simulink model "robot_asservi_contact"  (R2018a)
settings: Solver=VariableStepAuto  StartTime=0.0  StopTime=t(numel(t))  FixedStep=0.0001  RelTol=1e-3
model workspace: external: MATLAB File (data not in the file)
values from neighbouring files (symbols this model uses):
  D = [1500 1500 1000 0 0 0]    [TP_6Axes_main.m]
  dt = 0.01    [TP_6axes_trajectoire_polynomiale.m]    (also in TP_6axes_trajectoire_rectangulaire.m = 0.005)
  I = [0 0 0 0 0 0]    [TP_6Axes_main.m]
  mu = mu/3    [TP_6Axes_main.m]
  nx = length(ref)    [Jnum.m]    (also in TP_6axes_trajectoire_rectangulaire.m = 0.6)
  P = [16000 15000 14000 3000 3000 3000]    [TP_6Axes_main.m]
  q_targ = zeros(6,numel(p_targ(1,:)))    [TP_6axes_trajectoire_polynomiale.m]    (also in TP_6axes_trajectoire_rectangulaire.m)
  X = [T(1:3,4);Euler]    [MGD_6axes.m]    (also in TP_6axes_trajectoire_polynomiale.m = Trace_6axes_trajectoire(q_targ,p_targ,rob); TP_6axes_trajectoire_rectangulaire.m = Trace_6axes_trajectoire(q_targ,p_targ,rob); Trace_6axes.m = [0 0 0; Trace_6axes_trajectoire.m = [0 0 0)
undefined symbols (not defined in the file or in its folder): deg, kg, m, mm, N, rad, s, smiData, Y, Z
libraries: sm_lib x42, nesl_utility x23, Contact_Forces_Lib x1
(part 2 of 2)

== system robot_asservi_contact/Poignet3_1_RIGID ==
  ReferenceFrame : sm_lib/Frames and Transforms/Reference Frame
  Solid : sm_lib/Body Elements/Solid  InertiaType=Custom  Mass=smiData.Solid(2).mass  MassUnits=kg  CenterOfMass=smiData.Solid(2).CoM  CenterOfMassUnits=mm  MomentsOfInertia=smiData.Solid(2).MoI  MomentsOfInertiaUnits=kg*mm^2  ProductsOfInertia=smiData.Solid(2).PoI  ProductsOfInertiaUnits=kg*mm^2  DensityBased=on  Density=1000  DensityUnits=kg/m^3  DoExposeReferenceFrame=on  SerializedFrames=<Frames/>  GraphicType=FromGeometry  MarkerShape=Sphere  MarkerSize=10  GraphicVisPropType=SimpleVisualProperties  GraphicDiffuseColor=[0.4 1.0 1.0]  GraphicSpecularColor=[0.5 0.5 0.5 1.0]  GraphicAmbientColor=[0.15 0.15 0.15 1.0]  GraphicEmissiveColor=[0.0 0.0 0.0 1.0]  GraphicShininess=75  GraphicOpacity=smiData.Solid(2).opacity  GeometryShape=FromFile  RectangleSize=[1 1]  RectangleSizeUnits=m  BrickDimensions=[1 1 1]  BrickDimensionUnits=m  CylinderRadius=1  CylinderRadiusUnits=m  CylinderLength=1  CylinderLengthUnits=m  SphereRadius=1  SphereRadiusUnits=m  EllipsoidRadii=[1 1 1]  EllipsoidRadiiUnits=m  ExtrusionCrossSection=[1 1; -1 1; -1 -1; 1 -1]  ExtrusionCrossSectionUnits=m  ExtrusionLength=1  ExtrusionLengthUnits=m  PolygonNumSides=3  PolygonOuterRadius=1  PolygonOuterRadiusUnits=m  ExtGeomFileType=STL  ExtGeomFileName=Poignet3_Défaut_sldprt.STL  ExtGeomFileUnits=mm  RevolutionCrossSection=[1 1; 1 -1; 2 -1; 2 1]  RevolutionCrossSectionUnits=m  RevolutionExtent=Full  RevolutionAngle=180  RevolutionAngleUnits=deg
  Transform : sm_lib/Frames and Transforms/Rigid Transform  TranslationMethod=Cartesian  TranslationStandardOffset=0  TranslationLengthUnit=mm  TranslationStandardAxis=+Z  TranslationCartesianOffset=smiData.RigidTransform(6).translation  TranslationROffset=0  TranslationROffsetUnits=m  TranslationZOffset=0  TranslationZOffsetUnits=m  TranslationThetaOffset=0  TranslationThetaOffsetUnits=deg  RotationMethod=ArbitraryAxis  RotationAngleUnits=rad  RotationStandardAxis=+Z  RotationAngle=smiData.RigidTransform(6).angle  RotationArbitraryAxis=smiData.RigidTransform(6).axis  FollAlignAxisA=+X  BaseAlignAxisA=+Y  FollAlignAxisB=+Y  BaseAlignAxisB=+Z  RotationSequenceAxes=FollowerAxes  RotationSequence=XYX  RotationSequenceAngles=[0 0 0]  RotationSequenceAnglesUnits=deg  RotationMatrix=[1 0 0; 0 1 0; 0 0 1]
  F : PMIOPort  Side=Left
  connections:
  Solid/RConn1 -- ReferenceFrame/RConn1 -- Transform/LConn1
  Transform/RConn1 -- F/RConn1

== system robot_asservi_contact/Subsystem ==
  In1 : Inport
  Derivative : Derivative
  Derivative1 : Derivative
  Simulink-PS Converter6 : nesl_utility/Simulink-PS Converter  PhysicalDomain=network_engine_domain  SubClassName=ps_input  LeftPortType=input  RightPortType=output  PseudoPeriodic=off  Frequencies=[]  NoiseDistribution=none  NoiseParameters=[]  Unit=m  AffineConversion=off  FilteringAndDerivatives=provide  SimscapeFilterOrder=1  InputFilterTimeConstant=0.001  UdotUserProvided=2
  Conn1 : PMIOPort  Side=Right
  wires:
  In1/1 -> Derivative/1, Simulink-PS Converter6/1
  Derivative/1 -> Derivative1/1, Simulink-PS Converter6/2
  Derivative1/1 -> Simulink-PS Converter6/3
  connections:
  Simulink-PS Converter6/RConn1 -- Conn1/RConn1

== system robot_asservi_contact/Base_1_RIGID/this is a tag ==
  Transform : sm_lib/Frames and Transforms/Rigid Transform  TranslationMethod=Cartesian  TranslationStandardOffset=0  TranslationLengthUnit=mm  TranslationStandardAxis=+Z  TranslationCartesianOffset=smiData.RigidTransform(7).translation  TranslationROffset=0  TranslationROffsetUnits=m  TranslationZOffset=0  TranslationZOffsetUnits=m  TranslationThetaOffset=0  TranslationThetaOffsetUnits=deg  RotationMethod=ArbitraryAxis  RotationAngleUnits=rad  RotationStandardAxis=+Z  RotationAngle=smiData.RigidTransform(7).angle  RotationArbitraryAxis=smiData.RigidTransform(7).axis  FollAlignAxisA=+X  BaseAlignAxisA=+Y  FollAlignAxisB=+Y  BaseAlignAxisB=+Z  RotationSequenceAxes=FollowerAxes  RotationSequence=XYX  RotationSequenceAngles=[0 0 0]  RotationSequenceAnglesUnits=deg  RotationMatrix=[1 0 0; 0 1 0; 0 0 1]
  Transform2 : sm_lib/Frames and Transforms/Rigid Transform  TranslationMethod=Cartesian  TranslationStandardOffset=0  TranslationLengthUnit=mm  TranslationStandardAxis=+Z  TranslationCartesianOffset=smiData.RigidTransform(7).translation  TranslationROffset=0  TranslationROffsetUnits=m  TranslationZOffset=0  TranslationZOffsetUnits=m  TranslationThetaOffset=0  TranslationThetaOffsetUnits=deg  RotationMethod=ArbitraryAxis  RotationAngleUnits=rad  RotationStandardAxis=+Z  RotationAngle=smiData.RigidTransform(7).angle  RotationArbitraryAxis=smiData.RigidTransform(7).axis  FollAlignAxisA=+X  BaseAlignAxisA=+Y  FollAlignAxisB=+Y  BaseAlignAxisB=+Z  RotationSequenceAxes=FollowerAxes  RotationSequence=XYX  RotationSequenceAngles=[0 0 0]  RotationSequenceAnglesUnits=deg  RotationMatrix=[1 0 0; 0 1 0; 0 0 1]
  Conn1 : PMIOPort  Side=Left
  Conn2 : PMIOPort  Port=2  Side=Right
  Conn3 : PMIOPort  Port=3  Side=Left
  Conn4 : PMIOPort  Port=4  Side=Right
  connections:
  Conn1/RConn1 -- Transform/LConn1
  Transform/RConn1 -- Conn2/RConn1
  Transform2/LConn1 -- Conn3/RConn1
  Transform2/RConn1 -- Conn4/RConn1
